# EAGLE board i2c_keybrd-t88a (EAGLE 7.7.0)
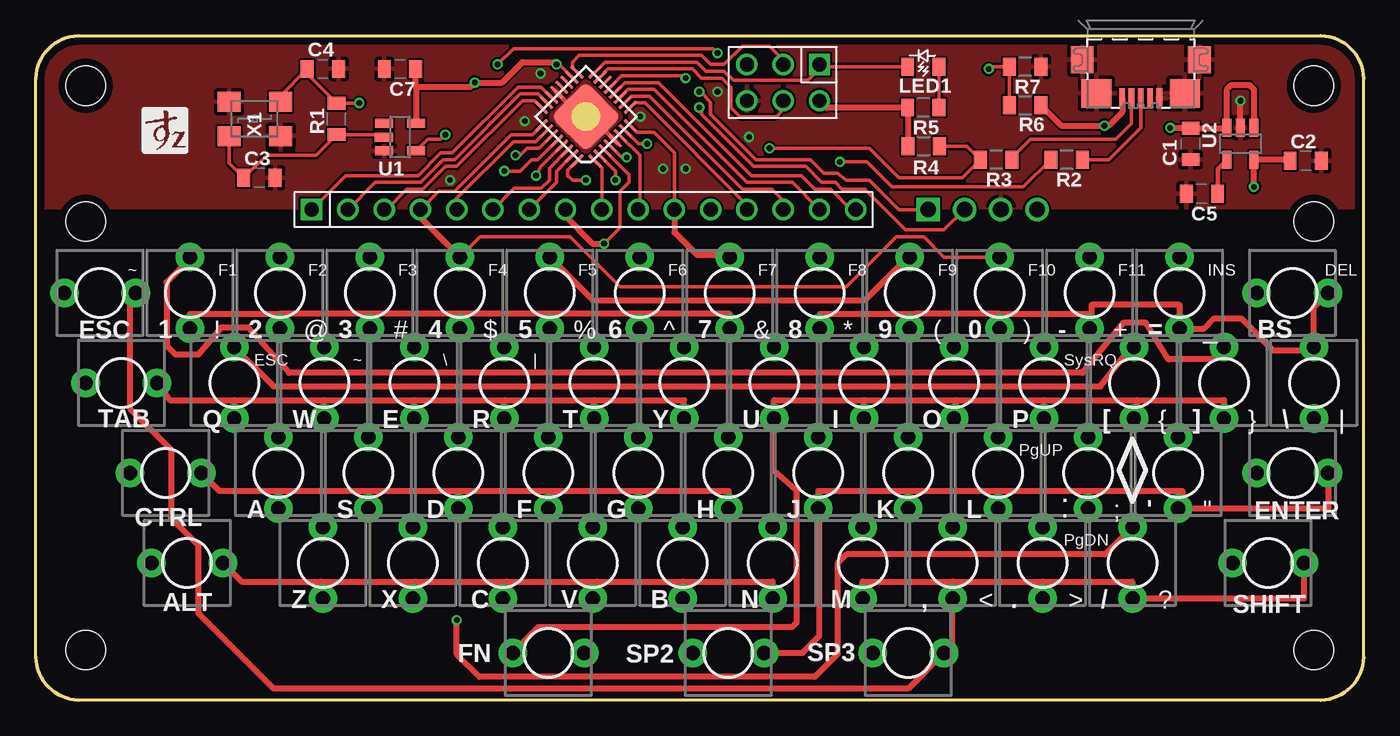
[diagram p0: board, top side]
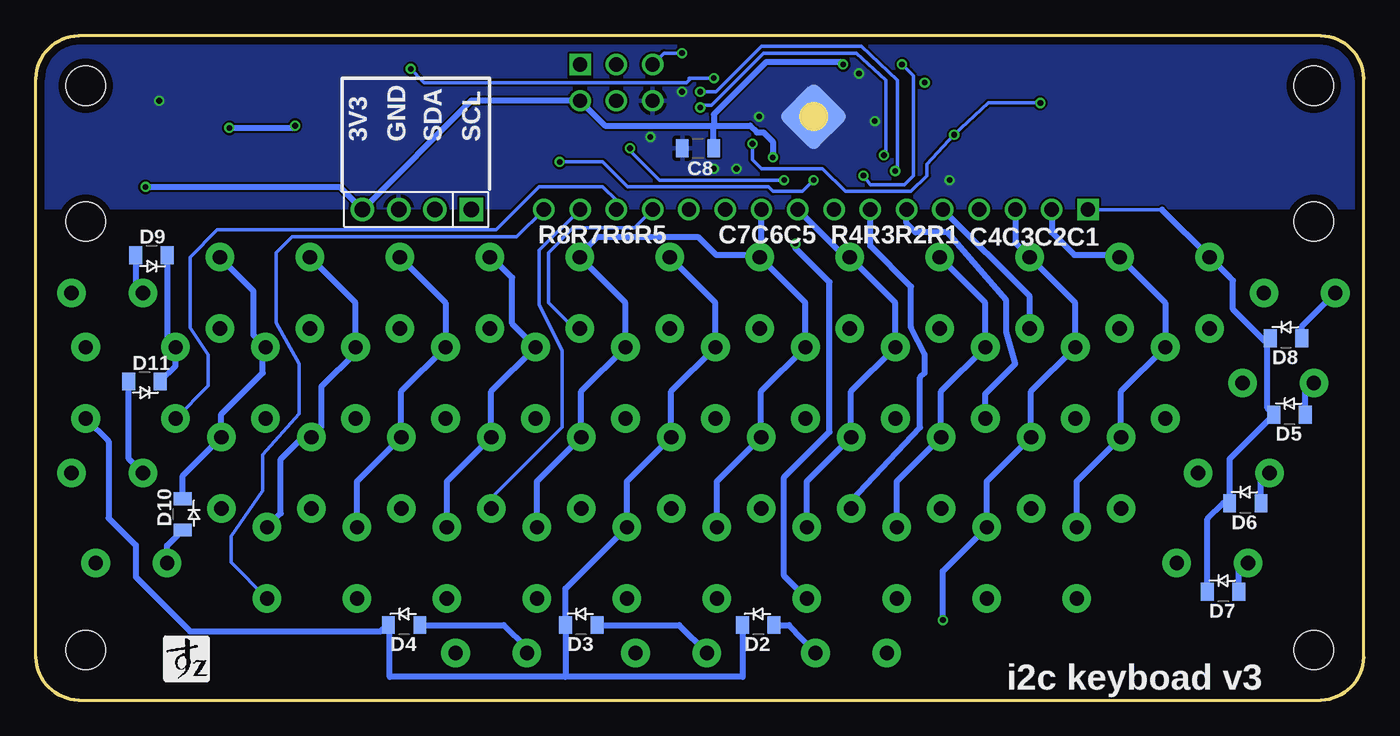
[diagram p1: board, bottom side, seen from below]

Size 93 x 46.5 mm. Coordinates in mm from the lower left corner, seen from the top.
Outline: 90,0 3,0 arc-87 0,3 0,43.5 arc-87 3,46.5 90,46.5 arc-87 93,43.5 93,3 arc-87 90,0
Copper layers (1*16): Top 0.035mm / dielectric 1.6mm / Bottom 0.035mm
Design rules "Elecrow_2-layer_PCB_eagle_rule": minimum track width 6mil, minimum drill 12mil, track to track 6mil, track to pad 6mil, pad to pad 6mil, via to via 8mil, smd to smd 0mil, copper to edge 20mil, drill to drill 10mil, minimum pad ring 6mil, minimum via ring 6mil, stop-mask expansion 0mil, vias tented up to drill 100mil, thermal gap 10mil
Holes 2.75 mm at 3.5,33.5 3.5,3.5 89.5,3.5 89.5,33.5 89.5,43 3.5,43

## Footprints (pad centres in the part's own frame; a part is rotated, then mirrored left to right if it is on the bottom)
TACTSW-2PIN = drill 1 pad 2: P$1 0,2.5; P$2 0,-2.5
C2012 = smd 0.9 x 1.25: 1 -1.1,0; 2 1.1,0
ZX62M = smd 1.35 x 0.4: 1 2.675,-1.3; 2 2.675,-0.65; 3 2.675,0; 4 2.675,0.65; 5 2.675,1.3 | smd 1.9 x 1.6: M1 0,-4.1; M2 0,4.1 | smd 2 x 2.1: M3 2.35,3.1; M4 2.35,-3.1
PINHDR2X3 = drill 1 square: 1 -2.54,-1.27 | drill 1: 2 -2.54,1.27; 3 0,-1.27; 4 0,1.27; 5 2.54,-1.27; 6 2.54,1.27
PINHDR1X4 = drill 1.1 square: 1 -3.81,0 | drill 1.1: 2 -1.27,0; 3 1.27,0; 4 3.81,0
PINHDR1X16_1.0 = drill 1 square: 1 -19.05,0 | drill 1: 2 -16.51,0; 3 -13.97,0; 4 -11.43,0; 5 -8.89,0; 6 -6.35,0; 7 -3.81,0; 8 -1.27,0; 9 1.27,0; 10 3.81,0; 11 6.35,0; 12 8.89,0; 13 11.43,0; 14 13.97,0; 15 16.51,0; 16 19.05,0
D2012 = smd 0.9 x 1.25: 1 -1.1,0; 2 1.1,0
LED2012 = smd 0.9 x 1.25: 1 -1.1,0; 2 1.1,0
R2012 = smd 0.9 x 1.25: 1 -1.1,0; 2 1.1,0
SOT235 = smd 0.635 x 1.27: 1 -0.95,-1.125; 2 0.013,-1.135; 3 0.95,-1.125; 4 0.95,1.125; 5 -0.95,1.125
QFN32 = smd 1.2 x 0.25: 1 -2.65,1.75; 2 -2.65,1.25; 3 -2.65,0.75; 4 -2.65,0.25; 5 -2.65,-0.25; 6 -2.65,-0.75; 7 -2.65,-1.25; 8 -2.65,-1.75; 17 2.65,-1.75; 18 2.65,-1.25; 19 2.65,-0.75; 20 2.65,-0.25; 21 2.65,0.25; 22 2.65,0.75; 23 2.65,1.25; 24 2.65,1.75 | smd 0.25 x 1.2: 9 -1.75,-2.65; 10 -1.25,-2.65; 11 -0.75,-2.65; 12 -0.25,-2.65; 13 0.25,-2.65; 14 0.75,-2.65; 15 1.25,-2.65; 16 1.75,-2.65; 25 1.75,2.65; 26 1.25,2.65; 27 0.75,2.65; 28 0.25,2.65; 29 -0.25,2.65; 30 -0.75,2.65; 31 -1.25,2.65; 32 -1.75,2.65 | smd 3.5 x 3.5: P$1 0,0 | smd 3.5 x 3.5 bottom: P$2 0,0
FA238 = smd 1.6 x 1.4: 1 -1.8,-1.2; 2 1.8,-1.2; 3 1.8,1.2; 4 -1.8,1.2

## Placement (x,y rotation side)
0  TACTSW22P  [TACTSW-2PIN]  67.5,28.5 0 top
1  TACTSW22P  [TACTSW-2PIN]  10.8,28.5 0 top
2  TACTSW22P  [TACTSW-2PIN]  17.1,28.5 0 top
3  TACTSW22P  [TACTSW-2PIN]  23.4,28.5 0 top
4  TACTSW22P  [TACTSW-2PIN]  29.7,28.5 0 top
5  TACTSW22P  [TACTSW-2PIN]  36,28.5 0 top
6  TACTSW22P  [TACTSW-2PIN]  42.3,28.5 0 top
7  TACTSW22P  [TACTSW-2PIN]  48.6,28.5 0 top
8  TACTSW22P  [TACTSW-2PIN]  54.9,28.5 0 top
9  TACTSW22P  [TACTSW-2PIN]  61.2,28.5 0 top
'  TACTSW22P  [TACTSW-2PIN]  80,15.9 0 top
,  TACTSW22P  [TACTSW-2PIN]  64.2,9.6 0 top
-  TACTSW22P  [TACTSW-2PIN]  73.8,28.5 0 top
.  TACTSW22P  [TACTSW-2PIN]  70.5,9.6 0 top
/  TACTSW22P  [TACTSW-2PIN]  76.8,9.6 0 top
=  TACTSW22P  [TACTSW-2PIN]  80.1,28.5 0 top
[  TACTSW22P  [TACTSW-2PIN]  76.9,22.2 0 top
\\  TACTSW22P  [TACTSW-2PIN]  89.5,22.2 0 top
]  TACTSW22P  [TACTSW-2PIN]  83.2,22.2 0 top
A  TACTSW22P  [TACTSW-2PIN]  17,15.9 0 top
ALT  TACTSW22P  [TACTSW-2PIN]  10.6,9.6 90 top
B  TACTSW22P  [TACTSW-2PIN]  45.3,9.6 0 top
BS  TACTSW22P  [TACTSW-2PIN]  88,28.5 90 top
C  TACTSW22P  [TACTSW-2PIN]  32.7,9.6 0 top
C1  10u  [C2012]  80.87,38.93 270 top
C2  10u  [C2012]  88.93,37.74 0 top
C3  22p  [C2012]  15.67,36.55 0 top
C4  22p  [C2012]  20.11,44.17 0 top
C5  0.01uF/NC  [C2012]  81.66,35.44 180 top
C6  MICRO-USBM  [ZX62M]  77.38,44.81 270 top
C7  1u  [C2012]  25.51,44.17 180 top
C8  1u  [C2012]  46.62,38.62 180 bottom
CLN  TACTSW22P  [TACTSW-2PIN]  73.7,15.9 0 top
CN1  PINHDR62X  [PINHDR2X3]  52.34,43.22 180 top
CN2  CONN4N  [PINHDR1X4]  66.31,34.33 180 bottom
CON1  PINHDR161  [PINHDR1X16_1.0]  38.37,34.33 0 top
CTRL  TACTSW22P  [TACTSW-2PIN]  9.1,15.9 90 top
D  TACTSW22P  [TACTSW-2PIN]  29.6,15.9 0 top
D2  D/SMD2012  [D2012]  42.4,5.25 180 bottom
D3  D/SMD2012  [D2012]  54.8,5.25 180 bottom
D4  D/SMD2012  [D2012]  67.2,5.25 180 bottom
D5  D/SMD2012  [D2012]  5.2,19.98 180 bottom
D6  D/SMD2012  [D2012]  8.3,13.77 180 bottom
D7  D/SMD2012  [D2012]  9.85,7.57 180 bottom
D8  D/SMD2012  [D2012]  5.44,25.32 180 bottom
D9  D/SMD2012  [D2012]  84.89,31.14 0 bottom
D10  D/SMD2012  [D2012]  82.7,13 90 bottom
D11  D/SMD2012  [D2012]  85.38,22.3 0 bottom
E  TACTSW22P  [TACTSW-2PIN]  26.5,22.2 0 top
ENTER  TACTSW22P  [TACTSW-2PIN]  88,15.9 90 top
ESC  TACTSW22P  [TACTSW-2PIN]  4.5,28.5 90 top
F  TACTSW22P  [TACTSW-2PIN]  35.9,15.9 0 top
FN  TACTSW22P  [TACTSW-2PIN]  35.9,3.3 270 top
G  TACTSW22P  [TACTSW-2PIN]  42.2,15.9 0 top
H  TACTSW22P  [TACTSW-2PIN]  48.5,15.9 0 top
I  TACTSW22P  [TACTSW-2PIN]  58,22.2 0 top
J  TACTSW22P  [TACTSW-2PIN]  54.8,15.9 0 top
K  TACTSW22P  [TACTSW-2PIN]  61.1,15.9 0 top
L  TACTSW22P  [TACTSW-2PIN]  67.4,15.9 0 top
LED1  D/SMDL  [LED2012]  62.16,44.33 180 top
M  TACTSW22P  [TACTSW-2PIN]  57.9,9.6 0 top
N  TACTSW22P  [TACTSW-2PIN]  51.6,9.6 0 top
O  TACTSW22P  [TACTSW-2PIN]  64.3,22.2 0 top
P  TACTSW22P  [TACTSW-2PIN]  70.6,22.2 0 top
Q  TACTSW22P  [TACTSW-2PIN]  13.9,22.2 0 top
R  TACTSW22P  [TACTSW-2PIN]  32.8,22.2 0 top
R1  1M  [R2012]  21.07,40.68 90 top
R2  22  [R2012]  72.18,37.82 180 top
R3  22  [R2012]  67.26,37.82 180 top
R4  1K5  [R2012]  62.18,38.77 0 top
R5  1K  [R2012]  62.16,41.47 180 top
R6  15K  [R2012]  69.28,41.63 0 top
R7  30K  [R2012]  69.28,44.33 180 top
S  TACTSW22P  [TACTSW-2PIN]  23.3,15.9 0 top
SHIFT  TACTSW22P  [TACTSW-2PIN]  86.3,9.6 90 top
SP2  TACTSW22P  [TACTSW-2PIN]  48.5,3.3 90 top
SP3  TACTSW22P  [TACTSW-2PIN]  61.1,3.3 90 top
T  TACTSW22P  [TACTSW-2PIN]  39.1,22.2 0 top
TAB  TACTSW22P  [TACTSW-2PIN]  6,22.2 90 top
U  TACTSW22P  [TACTSW-2PIN]  51.7,22.2 0 top
U1  1G14  [SOT235]  25.51,39.41 270 top
U2  TAR5SB  [SOT235]  84.36,38.93 180 top
U3  ATTINY88/TQFPQ  [QFN32]  38.53,40.84 135 top
V  TACTSW22P  [TACTSW-2PIN]  39,9.6 0 top
W  TACTSW22P  [TACTSW-2PIN]  20.2,22.2 0 top
X  TACTSW22P  [TACTSW-2PIN]  26.4,9.6 0 top
X1  16MHz  [FA238]  15.35,40.68 0 top
Y  TACTSW22P  [TACTSW-2PIN]  45.4,22.2 0 top
Z  TACTSW22P  [TACTSW-2PIN]  20.1,9.6 0 top

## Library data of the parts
0 1-9 ' , - . / = [ \\ ] A ALT B BS C C1-C8 CLN CN1 CN2 CON1 CTRL D D2-D11 E ENTER ESC F FN G H I J K L LED1 M N O P Q R R1-R7 S SHIFT SP2 SP3 T TAB U U1-U3 V W X X1 Y Z = SRT162-020

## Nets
5V: C1.1 C6.1 R6.2 U2.1 U2.3
COL1: 1.P$1 ].P$1 CON1.1 D5.2 D6.2 D7.2 D8.2 D9.2 D11.2 U3.22
COL2: 2.P$1 '.P$1 =.P$1 [.P$1 A.P$1 CON1.2 D10.2 Q.P$1 U3.23 Z.P$1
COL3: 3.P$1 -.P$1 /.P$1 CLN.P$1 CON1.3 P.P$1 S.P$1 U3.24 W.P$1 X.P$1
COL4: 0.P$1 4.P$1 ..P$1 C.P$1 CON1.4 D.P$1 E.P$1 L.P$1 O.P$1 U3.25
COL5: 5.P$1 9.P$1 ,.P$1 CON1.9 F.P$1 I.P$1 K.P$1 R.P$1 U3.1 V.P$1
COL6: 6.P$1 8.P$1 B.P$1 CON1.10 G.P$1 J.P$1 M.P$1 T.P$1 U3.6 U.P$1
COL7: 7.P$1 \\.P$2 CON1.11 D2.2 D3.2 D4.2 H.P$1 N.P$1 U3.8 Y.P$1
GND: C1.2 C2.2 C3.2 C4.2 C5.2 C6.5 C6.M1 C6.M2 C6.M3 C6.M4 C7.2 C8.2 CN1.6 CN2.3 R7.1 U1.3 U2.2 U3.5 U3.21 U3.P$1 U3.P$2 X1.2 X1.4
MISO: CN1.1 LED1.2 U3.16
MOSI: CN1.4 U3.15
N$1: D10.1 SHIFT.P$1
N$2: D3.1 SP2.P$1
N$3: D4.1 SP3.P$1
N$4: D2.1 FN.P$1
N$5: D5.1 TAB.P$1
N$6: CTRL.P$1 D6.1
N$7: ALT.P$1 D7.1
N$8: D8.1 ESC.P$1
N$9: D11.1 ENTER.P$1
N$10: BS.P$1 D9.1
N$11: LED1.1 R5.1
N$12: C5.1 U2.4
N$13: R6.1 R7.2 U3.13
N$14: R2.2 U3.32
N$15: C6.3 R2.1
N$16: C6.2 R3.1
N$17: R3.2 R4.2 U3.2
N$19: CN1.3 U3.17
N$31: U3.19
N$33: U3.20
ROW1: 1.P$2 2.P$2 3.P$2 4.P$2 5.P$2 6.P$2 7.P$2 CON1.5 U3.26
ROW2: CON1.6 E.P$2 Q.P$2 R.P$2 T.P$2 TAB.P$2 U3.30 W.P$2 Y.P$2
ROW3: A.P$2 CON1.7 CTRL.P$2 D.P$2 F.P$2 G.P$2 H.P$2 S.P$2 U3.31
ROW4: ALT.P$2 B.P$2 C.P$2 CON1.8 N.P$2 U3.3 V.P$2 X.P$2 Z.P$2
ROW5: 0.P$2 8.P$2 9.P$2 -.P$2 =.P$2 \\.P$1 BS.P$2 CON1.13 U3.9
ROW6: [.P$2 ].P$2 CON1.14 FN.P$2 I.P$2 O.P$2 P.P$2 U3.10 U.P$2
ROW7: '.P$2 CLN.P$2 CON1.15 ENTER.P$2 J.P$2 K.P$2 L.P$2 SP2.P$2 U3.11
ROW8: ,.P$2 ..P$2 /.P$2 CON1.16 ESC.P$2 M.P$2 SHIFT.P$2 SP3.P$2 U3.12
SCL: CN2.1 U3.28
SDA: CN2.2 U3.27
VOUT: C2.1 C7.1 C8.1 CN1.2 CN2.4 R4.1 R5.2 U1.5 U2.5 U3.4 U3.18
XIN: C3.1 R1.1 U1.2 X1.1
XOUT: C4.1 R1.2 U1.4 U3.7 X1.3
~RESET: CN1.5 U3.29

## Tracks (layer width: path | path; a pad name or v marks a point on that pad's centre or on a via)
5V  (via drill 0.4)
  Top 0.305: 79.45,40.03 v79.44,40.05 | 83.39,40.03 U2.3 | U2.1
  Top 0.406: 79.45,40.03 C1.1 83.39,40.03 | U2.3 83.41,42.75 83.72,43.06 85,43.06 85.31,42.74 U2.1 | C6.1 76.08,41.13 75.15,40.2 v74.83,40.2 71.81,40.2 R6.2
  Bottom 0.305: 74.99,40.05 v74.83,40.2
  Bottom 0.406: v79.44,40.05 74.99,40.05
COL1
  Top 0.254: U3.22 35.4,42.9 33.77,42.9 29.16,38.3 28.37,38.3 26.78,36.71 21.7,36.71 CON1.1
  Top 0.406: ].P$1 82.35,23.85 79.33,23.85 77.74,26.39 76.15,26.39 73.3,22.9 17.73,22.9 14.88,26.07 12.97,26.07 11.38,24.17 9.79,24.17 9.16,24.8 9.16,29.25 10.8,30.89 1.P$1
  Bottom 0.254: CON1.1 14.13,34.33
  Bottom 0.406: D7.2 10.95,12.68 9.85,13.77 D6.2 9.4,16.88 D5.2 6.75,20.43 6.75,25.12 | ].P$1 83.15,24.75 | D11.2 83.2,23.38 ].P$1 | D9.2 83.78,25.29 ].P$1 | 1.P$1 14.13,34.33 | 9.4,29.6 1.P$1 | 6.75,25.12 D8.2 | 6.75,25.12 6.93,25.12 9.16,27.34 9.16,29.36 1.P$1
COL2
  Top 0.254: U3.23 35.17,42.43 33.92,42.43 29.32,37.82 28.53,37.82 26.94,36.23 23.77,36.23 CON1.2
  Top 0.406: Q.P$1 16.65,21.95 74.56,21.95 76.68,24.7 [.P$1
  Bottom 0.406: CON1.2 21.86,32.74 20.27,31.16 17.25,31.16 2.P$1 13.9,27.8 Q.P$1 17,21.6 A.P$1 20.1,15.3 Z.P$1 | D10.2 82.7,15.7 '.P$1 80,20 77.11,22.9 77.11,23.85 76.79,24.17 76.79,24.59 [.P$1 77.74,25.54 77.74,28.61 80.1,30.98 =.P$1
COL3  (via drill 0.4)
  Top 0.254: U3.24 34.94,41.95 34.08,41.95 29.48,37.35 28.69,37.35 27.1,35.76 25.99,35.76 24.56,34.33 CON1.3
  Top 0.406: /.P$1 74.9,10.2 56.78,10.2 56.15,9.56 56.15,3.21 54.56,1.63 31.07,1.63 29.48,3.21 v29.48,5.6
  Bottom 0.406: CON1.3 24.4,32 3.P$1 20.2,27.8 W.P$1 23.3,21.6 S.P$1 26.4,15.3 X.P$1 | -.P$1 70.6,27.8 P.P$1 70.6,24.32 72.98,21.95 72.98,19.12 CLN.P$1 74.3,18.4 75.83,16.87 75.83,13.06 /.P$1 | 26.94,11.79 26.71,11.79 X.P$1 | v29.48,5.6 29.48,9.02 X.P$1
COL4
  Top 0.254: 4.P$1 31.12,32.42 37.42,32.42 40.91,28.93 56.78,28.93 60.28,32.42 62.18,32.42 63.61,31 0.P$1 | U3.25 34.78,39.57 33.29,39.57 29.32,35.6 28.21,35.6 CON1.4
  Top 0.406: 67.1,31 0.P$1 | 4.P$1 26.94,33.76 CON1.4
  Bottom 0.406: C.P$1 32.7,15.3 D.P$1 29.6,21.6 E.P$1 26.5,27.8 4.P$1 | 0.P$1 64.3,27.8 O.P$1 67.4,21.6 L.P$1 70.5,15.3 ..P$1
COL5
  Top 0.254: U3.1 39.64,37.25 CON1.9
  Top 0.406: 5.P$1 39.02,27.98 58.05,27.98 61.08,31 9.P$1
  Bottom 0.406: V.P$1 39,15.3 F.P$1 35.9,21.6 R.P$1 32.8,27.8 5.P$1 36.31,31 CON1.9 | ,.P$1 64.2,15.3 K.P$1 61.1,21.6 I.P$1 59.64,26.34 59.64,29.57 61.08,31 9.P$1
COL6
  Top 0.254: U3.6 42.3,38.13 42.3,34.45 CON1.10
  Bottom 0.406: M.P$1 57.9,15.3 J.P$1 54.8,21.6 U.P$1 51.7,27.8 8.P$1 54.9,31.13 53.61,32.42 46.62,32.42 45.35,31.16 42.45,31.16 6.P$1 | B.P$1 45.3,15.3 G.P$1 42.2,21.6 T.P$1 39.1,27.8 6.P$1 | 6.P$1 42.18,31.12 CON1.10
COL7
  Top 0.254: U3.8 42.12,39.73 43.29,39.73 44.72,38.3 CON1.11
  Top 0.406: CON1.11 44.72,32.74 46.31,31.16 48.45,31.16 7.P$1
  Bottom 0.406: 89.67,19.98 89.49,19.98 | 89.49,19.98 89.08,19.98 | D2.2 43.5,1.63 55.9,1.63 | 55.9,1.63 68.22,1.63 68.22,5.25 D4.2 68.4,5.25 68.85,4.8 82.19,4.8 86,8.61 86,10.84 87.9,12.74 87.9,18.1 \\.P$2 89.49,19.71 89.49,19.98 | 55.9,1.63 D3.2 55.9,7.8 N.P$1 51.6,15.3 H.P$1 48.5,21.6 Y.P$1 45.4,27.8 7.P$1
GND  (via drill 0.4)
  Top 0.305: U3.5 38.88,40.84 U3.P$2 38.17,40.84 U3.21 | 84.35,41.94 v84.36,41.95
  Top 0.406: U2.2 84.35,41.94
  other vias: 35.35,43.85 42.34,40.84 43.93,37.19 34.24,40.52 29,36.39 47.74,42.59 49.96,39.41 45.51,37.19
  pour Top: -4.02,50.2 95.52,50.52 97.74,34.5 -4.02,34.5 -4.33,50.36
  pour Bottom: 99.01,52.9 99.81,34.5 -5.6,34.5 -6.08,53.06
MISO
  Top 0.254: U3.16 39.86,44.65 46.31,44.65 46.94,44.01 48.21,44.01 48.85,43.38 54.09,43.38 54.88,44.17 CN1.1 55.04,44.33 LED1.2
MOSI
  Top 0.254: U3.15 40.09,44.17 45.99,44.17 46.62,43.54 48.05,43.54 48.69,42.9 48.69,41.47 49.32,40.84 51.86,40.84 52.34,41.31 CN1.4
N$1
  Bottom 0.406: SHIFT.P$1 83.8,10.8 D10.1
N$2
  Bottom 0.406: D3.1 47.95,5.25 SP2.P$1
N$3
  Bottom 0.406: D4.1 60.23,5.25 58.67,3.7 SP3.P$1
N$4
  Bottom 0.406: D2.1 40.25,5.25 FN.P$1
N$5
  Bottom 0.406: D5.1 4.1,21.6 TAB.P$1
N$6
  Bottom 0.406: D6.1 7.2,15.95 CTRL.P$1
N$7
  Bottom 0.406: D7.1 8.75,9.75 ALT.P$1
N$8
  Bottom 0.406: D8.1 4.34,26.16 ESC.P$1
N$9
  Bottom 0.406: ENTER.P$1 86.48,16.88 D11.1
N$10
  Bottom 0.406: D9.1 85.98,28.98 BS.P$1
N$11
  Top 0.254: LED1.1 R5.1
N$12
  Top 0.305: U2.4 82.76,37.14 C5.1
N$13  (via drill 0.4)
  Top 0.254: U3.13 41.03,43.7 45.35,43.7 v45.51,43.54 | R6.1 R7.2 66.9,44.33 v66.74,44.17
  Bottom 0.254: v45.51,43.54 47.1,43.54 | 47.1,43.54 47.26,43.54 | v66.74,44.17 65.79,43.22 47.42,43.22 47.1,43.54
N$14  (via drill 0.4)
  Top 0.254: U3.32 37.26,37.09 37.26,36.71 37.58,36.39 v38.53,36.39 | v56.31,37.66 58.21,37.66 59.96,35.92 69.18,35.92 R2.2
  Bottom 0.254: v56.31,37.66 53.29,37.66 51.55,35.92 41.7,35.92 41.39,35.6 39.32,35.6 v38.53,36.39
N$15
  Top 0.254: C6.3 77.38,40.05 75.15,37.82 R2.1
N$16
  Top 0.254: C6.2 76.72,40.35 75.63,39.25 69.64,39.25 68.36,37.97 R3.1
N$17  (via drill 0.4)
  Top 0.254: U3.2 40.59,37.01 v40.59,36.39 | v51.39,38.62 58.37,38.62 60.44,36.55 64.89,36.55 R3.2 65.21,38.77 R4.2
  Bottom 0.254: v40.59,36.39 49.32,36.39 51.39,38.46 v51.39,38.62
N$19
  Top 0.254: U3.17 37.58,44.27 37.58,44.65 38.05,45.12 46.62,45.12 47.26,44.49 48.21,44.49 49.48,45.76 51.39,45.76 52.34,44.81 CN1.3
ROW1
  Top 0.254: U3.26 35.02,39.09 33.45,39.09 29.48,35.12 CON1.5
  Top 0.406: 7.P$2 48.6,27.03 42.3,27.03 | 42.3,27.03 36,27.03 | 36,27.03 29.7,27.03 | 29.7,27.03 23.4,27.03 | 23.4,27.03 17.1,27.03 | 17.1,27.03 2.P$2 | 1.P$2 10.8,27.03 17.1,27.03 | 3.P$2 23.4,27.03 | 4.P$2 29.7,27.03 | 5.P$2 36,27.03 | 6.P$2 42.3,27.03
  Bottom 0.406: 3.P$2 23.4,28.25 CON1.5
ROW2
  Top 0.254: CON1.6 33.5,35.81 35.4,35.81 35.99,36.39 35.99,37.24 U3.30
  Top 0.406: TAB.P$2 9.39,21 13.9,21 | 13.9,21 20.2,21 | 20.2,21 26.5,21 | 26.5,21 32.8,21 | 32.8,21 39.1,21 | 39.1,21 45.4,21 Y.P$2 | Q.P$2 13.9,21 | W.P$2 20.2,21 | E.P$2 26.5,21 | R.P$2 32.8,21 | T.P$2 39.1,21
  Bottom 0.406: CON1.6 32.02,33.38 31.38,32.74 29.16,32.74 25.04,27.98 25.04,25.76 24.4,23.54 26.5,21.43 E.P$2
ROW3
  Top 0.254: U3.31 36.47,37.01 36.47,36.23 CON1.7
  Top 0.406: CTRL.P$2 12.86,14.64 16.78,14.64 | 16.78,14.64 23.13,14.64 | 23.13,14.64 29.8,14.64 | 36.15,14.64 42.18,14.64 | 42.18,14.64 48.53,14.64 48.5,14.61 H.P$2 | A.P$2 17,14.43 16.78,14.64 | S.P$2 23.3,14.48 23.13,14.64 | D.P$2 29.6,14.45 29.8,14.64 | G.P$2 42.2,14.62 42.18,14.64 | 29.8,14.64 36.15,14.64 | 36.15,14.64 36.15,13.4 F.P$2
  Bottom 0.406: F.P$2 35.9,13.94 31.07,19.09 31.07,22.58 30.75,22.9 30.75,24.17 31.7,26.07 31.7,28.93 34.56,31.79 CON1.7
ROW4  (via drill 0.4)
  Top 0.254: U3.3 41.55,36.76 41.55,36.23 40.91,35.6 40.91,33.06 v39.8,31.95
  Top 0.406: ALT.P$2 14.4,8.29 19.95,8.29 | 19.95,8.29 26.62,8.29 | 26.62,8.29 32.97,8.29 | 32.97,8.29 39.32,8.29 | 39.32,8.29 45.35,8.29 | 45.35,8.29 51.6,8.29 N.P$2 | B.P$2 45.35,7.15 45.35,8.29 | V.P$2 39.32,7.42 39.32,8.29 | C.P$2 32.7,8.02 32.97,8.29 | X.P$2 26.4,8.07 26.62,8.29 | Z.P$2 20.1,8.15 19.95,8.29 | CON1.8 37.1,33.85 39.01,31.95 v39.8,31.95
  Bottom 0.406: V.P$2 40.59,8.69 40.59,15.6 37.42,18.77 37.42,29.25 39.8,31.63 v39.8,31.95
ROW5
  Top 0.254: U3.9 41.96,41.79 42.66,41.79 49.8,34.65 CON1.13
  Top 0.406: 67.5,27.03 73.8,27.03 | 73.8,27.03 -.P$2 | 8.P$2 54.9,27.03 61.55,27.03 | 61.55,27.03 61.55,26 9.P$2 | 0.P$2 67.5,27.03 | 67.5,27.03 61.55,27.03 | 73.8,27.03 73.93,27.03 73.93,27.66 80.1,27.66 =.P$2 81.79,26 82.5,26.71 84.41,26.71 86.63,24.49 89.29,24.49 \\.P$1 89.5,27.5 BS.P$2
  Bottom 0.254: CON1.13 51.07,33.06 55.36,33.06 57.1,31.31 57.1,27.82 55.28,26
  Bottom 0.406: 55.28,26 8.P$2
ROW6
  Top 0.254: U3.10 41.73,42.27 42.97,42.27 49.48,35.76 51.55,35.76 52.34,34.97 CON1.14
  Top 0.406: FN.P$2 35.22,5.12 52.98,5.12 53.29,5.44 53.29,14.64 51.7,16.08 U.P$2 51.7,21 58,21 | 58,21 64.41,21 | 64.41,21 70.6,21 | 70.6,21 77.11,21 | 77.11,21 77.11,19.7 [.P$2 | I.P$2 58,21 | 64.41,21 64.41,19.7 O.P$2 | P.P$2 70.6,21 | 77.11,21 83.2,21 ].P$2
  Bottom 0.254: ].P$2 80.92,21.98 80.92,24.17 82.19,26.07 82.19,31 80.28,32.9 60.75,32.9 57.74,35.92 53.29,35.92 52.34,34.97 CON1.14
ROW7
  Top 0.254: U3.11 41.49,42.74 43.29,42.74 49.8,36.23 52.98,36.23 CON1.15
  Top 0.406: SP2.P$2 53.7,3.3 54.88,4.49 54.88,13.32 J.P$2 54.8,14.64 61.1,14.64 | K.P$2 61.1,14.64 | 61.1,14.64 67.4,14.64 | 67.4,14.64 73.7,14.64 | 73.7,14.64 80.28,14.64 80.28,13.4 '.P$2 90.5,13.4 ENTER.P$2 | L.P$2 67.4,14.64 | CLN.P$2 73.7,14.64
  Bottom 0.254: 61.1,14.14 56.15,19.09 56.15,24.49 57.74,27.66 57.74,31.47 CON1.15
  Bottom 0.406: K.P$2 61.1,14.14
ROW8
  Top 0.254: U3.12 41.26,43.22 43.61,43.22 50.12,36.71 53.61,36.71 54.56,35.76 55.67,35.76 57.1,34.33 CON1.16
  Top 0.406: 63.54,3.3 SP3.P$2 | M.P$2 57.9,8.29 64.2,8.29 | 64.2,8.29 70.5,8.29 | 70.5,8.29 76.79,8.29 76.79,7.1 /.P$2 88.8,7.1 SHIFT.P$2 | ..P$2 70.5,8.29 | 64.2,8.29 ,.P$2 64.2,3.9 SP3.P$2 | SP3.P$2 61.13,0.83 16.62,0.83 11.38,6.07 11.38,10.84 9.48,12.74 9.48,17.5 6.62,20.36 6.62,28.12 ESC.P$2
  Bottom 0.254: /.P$2 79.33,9.63 79.33,11.47 77.11,14.64 77.11,17.18 74.56,20.04 74.56,23.54 76.15,26.39 76.15,31.31 75.04,32.42 59.33,32.42 CON1.16
SCL  (via drill 0.4)
  Top 0.254: v46.47,42.59 46.62,42.59 47.26,41.79 47.26,41 50.44,37.82 54.24,37.82 55.2,36.87 56.15,36.87 56.78,36.39 58.37,36.39 60.44,34.33 CN2.1 | U3.28 35.16,37.82 34.72,37.82 33.92,37.03 v32.81,37.03
  Bottom 0.254: v32.81,37.03 32.66,37.19 32.66,43.38 35.2,45.76 42.18,45.76 45.35,42.59 v46.47,42.59
SDA  (via drill 0.4)
  Top 0.254: v46.47,41.47 46.62,41.31 46.62,41 50.28,37.35 53.93,37.35 55.04,36.23 55.99,36.23 56.47,35.76 58.05,35.76 60.91,32.9 63.61,32.9 CN2.2 | U3.27 35.25,38.62 34.4,38.62 33.92,38.14 v33.61,38.14
  Bottom 0.254: v33.61,38.14 33.45,38.3 33.45,43.38 35.51,45.28 42.02,45.28 45.67,41.63 46.31,41.63 v46.47,41.47
VOUT  (via drill 0.4)
  Top 0.254: v41.39,37.98 41.03,37.98 U3.4 | U3.18 36.78,44.35 v36.47,44.49 36.31,44.65 | 26.61,42.9 26.64,42.9
  Top 0.305: 87.7,37.81 C2.1
  Top 0.406: 36.31,44.65 34.08,44.65 32.66,43.22 v30.75,43.22 30.43,42.9 26.64,42.9 U1.5 | 87.7,37.81 U2.5 85.31,36.87 v85.31,35.92 | 61.23,41.54 61.23,41.47 61.21,41.45 61.08,41.45 | 26.61,42.9 C7.1 | 61.08,41.45 R5.2 | CN1.2 55.38,41.45 61.08,41.45 | 61.08,41.45 R4.1
  Bottom 0.254: v36.47,44.49 36.62,44.65
  Bottom 0.406: 45.51,40.2 53.13,40.2 CN1.2 62.5,41.95 CN2.4 71.71,35.92 v85.31,35.92 | 45.51,40.2 42.97,40.2 42.5,39.73 42.02,39.73 41.39,39.09 41.39,38.3 v41.39,37.98 | 36.62,44.65 41.86,44.65 45.51,41 45.51,40.2 | C8.1 45.52,40.19 45.51,40.2
XIN
  Top 0.254: X1.1 13.55,37.57 C3.1 16.16,38.14 19.64,38.14 R1.1 24.19,39.58 U1.2
XOUT  (via drill 0.4)
  Top 0.254: U3.7 42.2,38.93 v42.81,38.93 | X1.3 17.15,42.31 C4.1 19.01,43.83 R1.2 v22.64,41.78 v22.65,41.79 | v28.69,39.57 28.37,39.25 27.43,39.25 U1.4
  Bottom 0.254: v42.81,38.93 42.81,37.82 42.18,37.19 37.89,37.19 36.31,35.6 31.7,35.6 30.59,36.71 30.59,37.51 v28.69,39.57 26.3,41.79 v22.65,41.79
~RESET  (via drill 0.4)
  Top 0.254: U3.29 35.35,37.31 v35.04,36.71 | v32.34,44.49 33.45,45.6 47.42,45.6 v47.74,45.28
  Bottom 0.254: v35.04,36.71 34.56,36.08 32.18,36.08 31.54,36.71 31.54,43.7 v32.34,44.49 | CN1.5 49.01,45.28 v47.74,45.28

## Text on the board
tPlace: ~ | F1 | F2 | F3 | F4 | F5 | F6 | F7 | F8 | F9 | F10 | F11 | INS | DEL | ! | @ | # | $ | % | ^ | & | * | ( | ) | + | _ | ESC | ~ | \\ | | | SysRQ | { | } | | | PgUP | : | ; | " | PgDN | < | > | ?
bPlace: SCL | SDA | GND | 3V3 | C4C3C2C1 | R4R3R2R1 | C7C6C5 | R8R7R6R5 | i2c keyboad v3
Measures: 37mm | 46.5mm | 6.3mm pitch 2pin TACTSW board | 93mm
